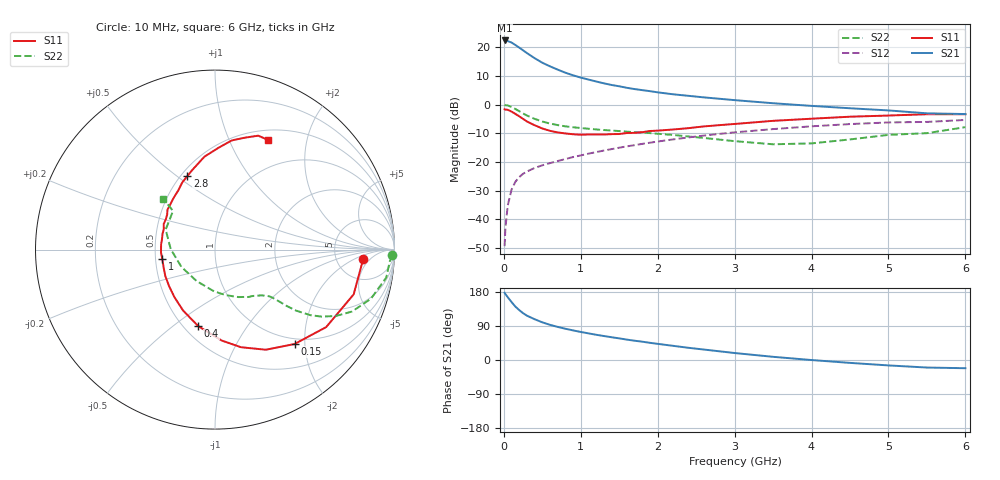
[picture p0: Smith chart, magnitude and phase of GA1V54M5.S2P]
! Infineon Technologies  Discrete & RF Semiconductors
! BF775
! Si NPN RF Bipolar Junction Transistor in SOT23
! VCE = 1.5 V  IC = 4.5 mA
! Common Emitter S-Parameters:  May  1996
# GHz  S  MA  R  50
!  f  S11  S21  S12  S22
! GHz  MAG  ANG  MAG  ANG  MAG  ANG  MAG  ANG
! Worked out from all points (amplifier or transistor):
!   36 points, 10 MHz to 6 GHz, reference 50 ohm
!   highest |S21| = 22.4 dB at 10 MHz (marker M1)
!   |S21| within 3 dB of that: start of sweep to 226.7 MHz
!   unconditionally stable (mu >= 1): 776.1 MHz to 4.367 GHz; 5.066 GHz to end of sweep
!   at 250 MHz: K = 0.47, MSG = 21.5 dB, |S12| = -24.1 dB
!   at 1.4 GHz: K = 1.16, MAG = 8.8 dB, |S12| = -15.5 dB
!   at 6 GHz: K = 1.01, MAG = 0.5 dB, |S12| = -5.4 dB
!   S11 on the Smith chart (normalised r, x): 10 MHz: 10, -3; 150 MHz: 0.90, -1.79; 400 MHz: 0.59, -0.62; 1 GHz: 0.54, -0.06; 2.8 GHz: 0.54, +0.55; 6 GHz: 0.62, +1.40
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0.01  0.8274 -3.6  13.13 177.4  0.0034 89.1  0.9894 -1.8
0.02  0.8184 -7.4  13.01 174.1  0.0069 88.3  0.9765 -3.7
0.05  0.8119 -17.9  12.8 165.9  0.0172 80.4  0.9667 -9.3
0.1  0.7549 -34.9  12.07 153.0  0.0328 71.9  0.9109 -17.5
0.15  0.6879 -49.9  10.94 140.9  0.0451 65.0  0.8382 -24.3
0.2  0.6256 -63.1  9.851 131.7  0.0545 60.7  0.7682 -28.8
0.25  0.5628 -75.1  8.834 123.5  0.0621 56.8  0.7005 -32.2
0.3  0.508 -85.8  7.909 117.0  0.0681 55.0  0.645 -34.5
0.4  0.4364 -102.4  6.448 107.6  0.0785 52.6  0.5642 -37.0
0.5  0.3833 -117.6  5.371 99.4  0.0874 51.6  0.5067 -38.2
0.6  0.3489 -130.2  4.642 92.8  0.0954 51.9  0.4669 -38.8
0.8  0.314 -151.6  3.595 82.5  0.1124 52.3  0.4173 -39.9
1  0.2983 -169.7  2.958 74.0  0.1299 52.8  0.3903 -41.4
1.1  0.3013 -177.0  2.73 70.3  0.1395 53.0  0.3793 -42.7
1.3  0.3009 169.1  2.349 63.3  0.1581 52.9  0.3602 -45.0
1.6  0.3195 153.4  1.961 53.8  0.1869 52.2  0.337 -49.9
2.2  0.3678 129.1  1.512 37.4  0.2474 48.0  0.2957 -63.5
2.8  0.4378 110.5  1.264 23.0  0.3081 42.0  0.2455 -83.4
3.5  0.521 96.5  1.056 8.4  0.374 33.3  0.2032 -120.2
4.5  0.615 81.3  0.863 -7.6  0.4574 20.2  0.2468 179.3
5.5  0.6789 69.2  0.704 -19.9  0.4986 5.8  0.3177 137.4
6  0.6787 64.4  0.684 -21.7  0.5398 1.8  0.4042 135.4
